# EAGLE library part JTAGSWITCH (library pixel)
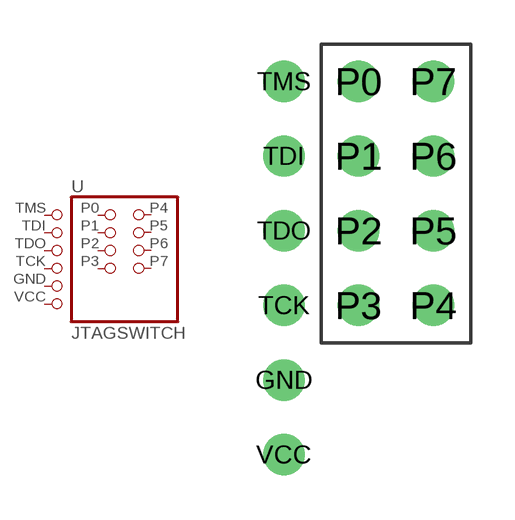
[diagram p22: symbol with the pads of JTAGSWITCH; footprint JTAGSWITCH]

Designator prefix -

## JTAGSWITCH  [JTAGSWITCH]
GND  GND  pas
P0  P0  pas
P1  P1  pas
P2  P2  pas
P3  P3  pas
P4  P4  pas
P5  P5  pas
P6  P6  pas
P7  P7  pas
TCK  TCK  pas
TDI  TDI  pas
TDO  TDO  pas
TMS  TMS  pas
VCC  VCC  pas

## Footprint JTAGSWITCH (pad centres in mm)
drill 0.9 pad 1.27: GND -3.81,-6.35; P0 -1.27,3.81; P1 -1.27,1.27; P2 -1.27,-1.27; P3 -1.27,-3.81; P4 1.27,-3.81; P5 1.27,-1.27; P6 1.27,1.27; P7 1.27,3.81; TCK -3.81,-3.81; TDI -3.81,1.27; TDO -3.81,-1.27; TMS -3.81,3.81; VCC -3.81,-8.89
